{attribute 'TcGenerated'}
{attribute 'no-analysis'}
{attribute 'linkalways'}
// This function has been automatically generated from the project information.
VAR_GLOBAL CONSTANT
	{attribute 'const_non_replaced'}
	stLibVersion_PMCLib : ST_LibVersion := (iMajor := 4, iMinor := 1, iBuild := 1, iRevision := 0, nFlags := 0, sVersion := '4.1.1');
END_VAR
